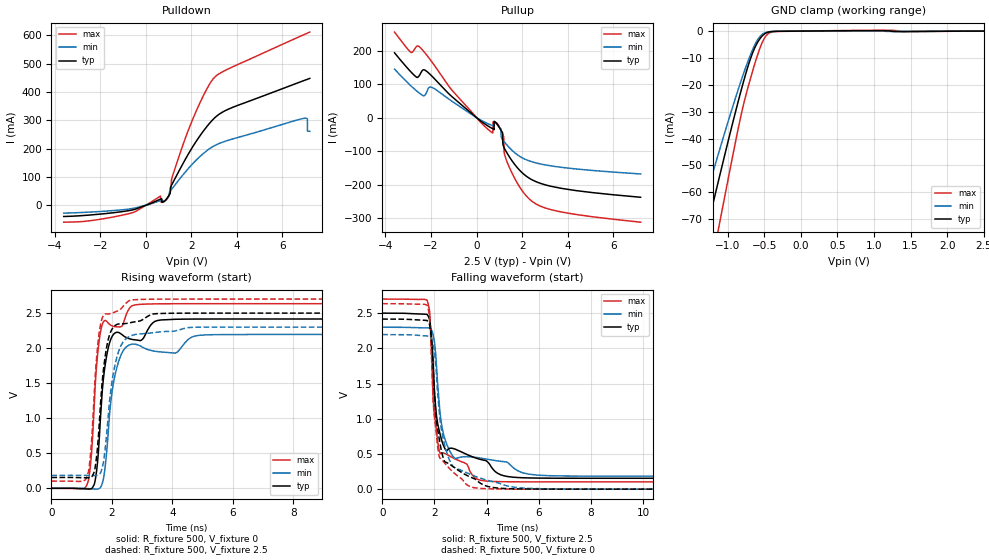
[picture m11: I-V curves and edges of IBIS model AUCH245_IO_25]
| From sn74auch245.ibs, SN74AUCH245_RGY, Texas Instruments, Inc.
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[Model]   AUCH245_IO_25
Model_type  3-state
Enable   Active-Low
Vref =   0
Rref =   500
Cref =   30p
Vmeas =   1.25
| variable   typ   min   max
C_comp   6.80pF   5.98pF   7.34pF
| C_pullup   8.70pF   3.80pF   12.73pF
| C_pulldown   8.07pF   6.10pF   17.07pF
| C_tri-state   6.80pF   5.98pF   7.34pF
[Temperature Range]   40   100   -40
| Ambient temperature   25   85   -40
[Voltage range]   2.5   2.3   2.7
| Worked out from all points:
|   slope of the pulldown table from 0 to 0.375 V, typ, clamps not added: 30.9 ohm
|   slope of the pullup table from 0 to 0.375 V, typ, clamps not added: 19.3 ohm
|   GND clamp passes 1 mA (typ) near -0.49 V on its own axis
|   rising waveform, R_fixture 500, V_fixture 0: 20-80 % time 299ps typ, 376ps min, 249ps max; typ from 0 V to 2.42 V
|   falling waveform, R_fixture 500, V_fixture 2.5: 20-80 % time 430ps typ, 451ps min, 285ps max; typ from 2.5 V to 0.155 V
|   rising waveform, R_fixture 500, V_fixture 2.5: 20-80 % time 302ps typ, 381ps min, 249ps max; typ from 0.154 V to 2.5 V
|   falling waveform, R_fixture 500, V_fixture 0: 20-80 % time 382ps typ, 497ps min, 290ps max; typ from 2.42 V to 0 V
[GND Clamp]
| AUCH245_IO_25
|   Voltage   I(typ)   I(min)   I(max)
-3.6V     -348.4mA   -291.7mA   -422.1mA
-1.435V   -91.27mA   -74.59mA   -117.4mA
-1.385V   -85.45mA   -69.82mA   -110.3mA
-1.285V   -73.88mA   -60.35mA   -96.12mA
-1.24V    -68.71mA   -56.13mA   -89.75mA
-1.115V   -54.48mA   -44.57mA   -72.08mA
-835mV    -23.98mA   -19.98mA   -33.54mA
-710mV    -12.03mA   -10.29mA   -19.72mA
-610mV    -5.111mA   -4.116mA   -10.43mA
-495mV    -1.031mA   -670.5uA   -2.519mA
-320mV    -85.07uA   -63.27uA   -141.3uA
2.5V      1.615nA    801.5nA    -13.03nA
[Pulldown]
| AUCH245_IO_25
|   Voltage   I(typ)   I(min)   I(max)
-3.6V     -39.47mA   -27.63mA   -59.61mA
-1.05V    -22.47mA   -15.92mA   -35.12mA
645mV     21.78mA    16.54mA    32.6mA
655mV     22.14mA    16.85mA    12.29mA
895mV     20.36mA    20.87mA    18.59mA
1.11V     67.72mA    53.86mA    54.57mA
1.88V     182.5mA    130.9mA    267.3mA
2.97V     304.5mA    208.5mA    447.6mA
6.945V    440.7mA    307.2mA    602.8mA
7.095V    445.1mA    304.6mA    608.1mA
7.1V      445.3mA    261.9mA    608.3mA
7.2V      448.2mA    261.3mA    611.8mA
[Pullup]
| AUCH245_IO_25
|   Voltage   I(typ)   I(min)   I(max)
-3.6V     193.8mA    145mA      255.7mA
-2.88V    136.6mA    94.91mA    194.8mA
-2.445V   133.8mA    70mA       207.7mA
-1.95V    123.4mA    90.09mA    165.6mA
450mV     -22.92mA   -16.7mA    -31.9mA
925mV     -21.65mA   -22.49mA   -18.57mA
1.14V     -45.38mA   -65.85mA   -48.65mA
1.185V    -86.11mA   -69.78mA   -56.17mA
1.215V    -91.01mA   -72.34mA   -105.6mA
1.435V    -116.7mA   -89.5mA    -148mA
2.43V     -185.7mA   -132mA     -250mA
7.2V      -238.1mA   -168.4mA   -312.5mA
[Ramp]
| AUCH245_IO_25
| variable   typ   min   max
dV/dt_r   1.46/3.04E-10   1.32/3.80E-10   1.59/2.50E-10
dV/dt_f   1.41/4.31E-10   1.27/4.58E-10   1.56/2.88E-10
R_load = 500
[Rising Waveform]
| AUCH245_IO_25
R_fixture =   500
C_fixture =   0
L_fixture =   0
V_fixture =   0
V_fixture_min = 0
V_fixture_max = 0
|   Time   V(typ)   V(min)   V(max)
0s        15.38nV    49.28nV    1.37nV
1.22ns    -10.92mV   -3.818mV   105.3mV
1.455ns   132.2mV    -11.16mV   1.516V
1.625ns   1.023V     11.16mV    2.235V
1.755ns   1.69V      230mV      2.391V
1.98ns    2.143V     1.292V     2.323V
2.305ns   2.202V     1.905V     2.307V
2.765ns   2.118V     2.056V     2.617V
4.105ns   2.412V     1.929V     2.634V
34.99ns   2.416V     2.195V     2.634V
[Falling Waveform]
| AUCH245_IO_25
R_fixture =   500
C_fixture =   0
L_fixture =   0
V_fixture =   2.5
V_fixture_min = 2.3
V_fixture_max = 2.7
|   Time   V(typ)   V(min)   V(max)
0s        2.5V       2.3V       2.7V
1.715ns   2.483V     2.29V      2.686V
1.82ns    2.397V     2.288V     2.494V
2ns       1.398V     2.089V     1.059V
2.195ns   812.7mV    1.167V     531.4mV
2.37ns    598.7mV    748.1mV    511mV
2.72ns    577.5mV    462.2mV    442.3mV
3.8ns     419mV      439.2mV    124.3mV
5.62ns    159.6mV    212.8mV    103.8mV
34.99ns   154.5mV    184.2mV    103.2mV
[Rising Waveform]
| AUCH245_IO_25
R_fixture =   500
C_fixture =   0
L_fixture =   0
V_fixture =   2.5
V_fixture_min = 2.3
V_fixture_max = 2.7
|   Time   V(typ)   V(min)   V(max)
0s        154.5mV    184.1mV    103.2mV
1.195ns   150.3mV    183mV      193.1mV
1.315ns   159.8mV    182mV      602.1mV
1.44ns    281.6mV    182.4mV    1.542V
1.62ns    1.186V     216.2mV    2.328V
1.755ns   1.811V     478.5mV    2.482V
1.94ns    2.211V     1.313V     2.491V
2.225ns   2.345V     1.956V     2.534V
2.62ns    2.364V     2.174V     2.684V
34.99ns   2.5V       2.3V       2.7V
[Falling Waveform]
| AUCH245_IO_25
R_fixture =   500
C_fixture =   0
L_fixture =   0
V_fixture =   0
V_fixture_min = 0
V_fixture_max = 0
|   Time   V(typ)   V(min)   V(max)
0s        2.416V     2.195V     2.634V
1.715ns   2.396V     2.175V     2.614V
1.82ns    2.324V     2.168V     2.424V
1.915ns   1.998V     2.115V     1.605V
1.99ns    1.432V     1.981V     1.056V
2.185ns   711.5mV    1.103V     462.9mV
2.645ns   338.6mV    359.9mV    266.7mV
3.505ns   151.5mV    191.3mV    22.11mV
6.225ns   1.128mV    4.699mV    274.3uV
34.99ns   51.27uV    53.67uV    12.92uV
